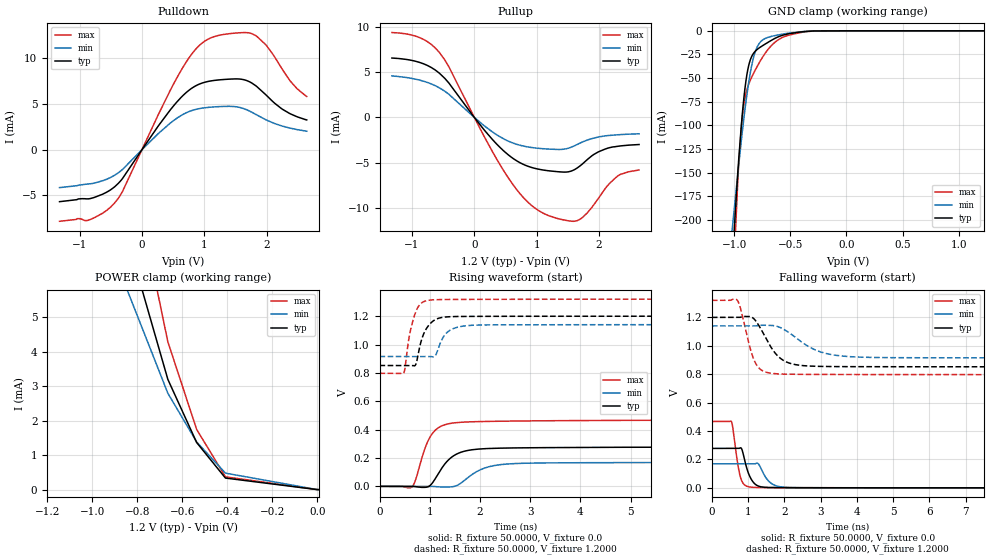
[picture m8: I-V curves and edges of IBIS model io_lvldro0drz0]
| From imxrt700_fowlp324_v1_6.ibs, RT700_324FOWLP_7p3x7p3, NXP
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[Model] io_lvldro0drz0
|   Model io_lvldro0drz0
| This model was characterised for following simulation conditions:
| External (pad) voltage:
|   - Typ: 1.2V,   - Min: 1.14V,   - Max: 1.32V
| Library cells for typ/min/max conditions are connected as defined below:
|  ipp_io - External Pad
|  ipp_do - Core Input
|  ipp_obe - Output Buffer Enable
|  config1v21v8 - vdd
|  drive0 - gnde
|  drive1 - gnde
|  gnd - gnd
|  gnde - gnde
|  ncgather - NC
|  vdd - vdd
|  vdde1v8 - vdde1v8
| All other pins connected to ground
Model_type I/O
Polarity   Non-Inverting
Enable   Active-Low
Vinl =   0.3600V
Vinh =   0.8400V
Vmeas =  0.6000V
Cref =   30.0000pF
Rref =   1.0000M
Vref =   1.2000V
C_comp   2.6161pF   2.5654pF   2.7101pF
|C_comp_pullup   1.3388pF   1.3968pF   1.2799pF
|C_comp_pulldown   0.0F   0.0F   0.0F
[Model Spec]
| variable   typ   min   max
Vinh   0.8400V   NA   NA
Vinl   0.3600V   NA   NA
Vref   1.8000V   1.8000V   1.8000V
Cref   30.0000pF   30.0000pF   30.0000pF
Rref   1.0000M   1.0000M   1.0000M
[Temperature Range]   25.0000   0.1250k   -40.0000
[Voltage Range]   1.2000V   1.1400V   1.3200V
[Pullup Reference]   1.2000V   1.1400V   1.3200V
[Pulldown Reference]   0.0V   0.0V   0.0V
[POWER Clamp Reference]   1.2000V   1.1400V   1.3200V
[GND Clamp Reference]   0.0V   0.0V   0.0V
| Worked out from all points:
|   slope of the pulldown table from 0 to 0.18 V, typ, clamps not added: 101 ohm
|   slope of the pullup table from 0 to 0.18 V, typ, clamps not added: 115 ohm
|   GND clamp passes 1 mA (typ) near -0.39 V on its own axis
|   POWER clamp passes 1 mA (typ) near -0.49 V on its own axis
|   rising waveform, R_fixture 50.0000, V_fixture 0.0: 20-80 % time 394ps typ, 485ps min, 296ps max; typ from 0 V to 0.278 V
|   rising waveform, R_fixture 50.0000, V_fixture 1.2000: 20-80 % time 204ps typ, 220ps min, 175ps max; typ from 0.852 V to 1.2 V
|   falling waveform, R_fixture 50.0000, V_fixture 0.0: 20-80 % time 218ps typ, 268ps min, 166ps max; typ from 0.278 V to 0 V
|   falling waveform, R_fixture 50.0000, V_fixture 1.2000: 20-80 % time 521ps typ, 847ps min, 323ps max; typ from 1.2 V to 0.852 V
[Pulldown]
|Voltage   I(typ)   I(min)   I(max)
-1.32V    -5.688mA   -4.151mA   -7.836mA
-856mV    -5.378mA   -3.749mA   -7.707mA
-440mV    -4.076mA   -2.805mA   -5.848mA
-312mV    -3.159mA   -2.166mA   -4.577mA
624mV     5.702mA    3.731mA    8.647mA
856mV     6.973mA    4.402mA    10.96mA
1.064V    7.478mA    4.635mA    12.12mA
1.568V    7.735mA    4.622mA    12.8mA
1.832V    6.962mA    3.837mA    12.46mA
1.992V    5.967mA    3.257mA    11.43mA
2.256V    4.407mA    2.573mA    8.725mA
2.64V     3.256mA    2.027mA    5.833mA
[Pullup]
|Voltage   I(typ)   I(min)   I(max)
-1.32V    6.575mA    4.592mA    9.394mA
-880mV    6.098mA    4.136mA    8.849mA
-560mV    4.9mA      3.277mA    7.198mA
-408mV    3.813mA    2.567mA    5.622mA
496mV     -3.862mA   -2.465mA   -6.171mA
792mV     -5.22mA    -3.183mA   -8.915mA
1.064V    -5.782mA   -3.445mA   -10.46mA
1.464V    -6.056mA   -3.485mA   -11.4mA
1.648V    -5.607mA   -3.003mA   -11.44mA
1.976V    -3.863mA   -2.192mA   -9.092mA
2.304V    -3.195mA   -1.922mA   -6.453mA
2.64V     -3.006mA   -1.816mA   -5.825mA
[GND_clamp]
|Voltage   I(typ)   I(min)   I(max)
-1.32V    -824mA     -526.2mA   -1.227A
-1.032V   -269.6mA   -225.5mA   -323.8mA
-968mV    -148.5mA   -150.4mA   -156.4mA
-936mV    -98.26mA   -114.7mA   -100.6mA
-920mV    -77.35mA   -98.01mA   -82.61mA
-880mV    -41.26mA   -61.23mA   -59.24mA
-856mV    -30.33mA   -43.55mA   -51.86mA
-816mV    -21.94mA   -23.19mA   -42.16mA
-744mV    -15.43mA   -9.413mA   -27.16mA
-584mV    -5.259mA   -3.813mA   -7.801mA
-352mV    -567.9uA   -545.2uA   -812.4uA
1.224V    19.17nA    663.1nA    12.5nA
[POWER_clamp]
|Voltage   I(typ)   I(min)   I(max)
-1.32V    19.77mA    14.89mA    27.18mA
-1.048V   11.92mA    9.166mA    16.41mA
-664mV    3.199mA    2.796mA    4.29mA
-536mV    1.366mA    1.383mA    1.747mA
-408mV    334.7uA    478.1uA    371.6uA
0V        17.28nA    129.7nA    13.53nA
8mV       16.9nA     117.4nA    13.43nA
[Ramp]
| variable   typ   min   max
dV/dt_r  0.1666/0.3936n   0.1014/0.4848n   0.2804/0.2955n
dV/dt_f  0.2087/0.5209n   0.1348/0.8462n   0.3138/0.3229n
R_load = 50.0000
[Rising Waveform]
R_fixture= 50.0000
V_fixture= 0.0
V_fixture_min= 0.0
V_fixture_max= 0.0
|time   V(typ)   V(min)   V(max)
0s        36.99nV    2.153uV    4.325nV
636.3ps   8.785uV    834.1nV    -6.706mV
715.1ps   -2.216mV   1.884uV    43.01mV
943.3ps   -5.366mV   -10.28uV   302.9mV
1.11ns    54.19mV    -1.954mV   395.8mV
1.474ns   215.3mV    -1.494mV   447mV
2.012ns   263.9mV    117.9mV    456.9mV
2.619ns   270.6mV    159.4mV    460.2mV
4.852ns   275.6mV    167.5mV    465.2mV
60ns      277.6mV    169.1mV    467.3mV
[Rising Waveform]
R_fixture= 50.0000
V_fixture= 1.2000
V_fixture_min= 1.1400
V_fixture_max= 1.3200
|time   V(typ)   V(min)   V(max)
0s        852.1mV    915.3mV    797mV
479.4ps   852.1mV    915.3mV    797.3mV
606.4ps   852.1mV    915.3mV    1.084V
741.2ps   881.8mV    915.3mV    1.247V
903.3ps   1.094V     915.3mV    1.306V
1.085ns   1.17V      913.6mV    1.315V
1.17ns    1.185V     971.1mV    1.317V
1.448ns   1.197V     1.109V     1.318V
2.199ns   1.199V     1.139V     1.319V
60ns      1.2V       1.14V      1.32V
[Falling Waveform]
R_fixture= 50.0000
V_fixture= 0.0
V_fixture_min= 0.0
V_fixture_max= 0.0
|time   V(typ)   V(min)   V(max)
0s        277.6mV    169.1mV    467.3mV
535.8ps   277.6mV    169.1mV    468.4mV
573.6ps   277.6mV    169mV      430mV
725.7ps   277.2mV    169mV      150mV
809.7ps   279.2mV    169mV      57.82mV
1.015ns   98.54mV    169mV      7.515mV
1.21ns    22.59mV    171.2mV    2.998mV
1.659ns   1.997mV    27.97mV    1.835mV
2.324ns   979.9uV    1.503mV    1.301mV
60ns      245.3nV    3.818uV    27.38nV
[Falling Waveform]
R_fixture= 50.0000
V_fixture= 1.2000
V_fixture_min= 1.1400
V_fixture_max= 1.3200
|time   V(typ)   V(min)   V(max)
0s        1.2V       1.14V      1.32V
697.5ps   1.2V       1.14V      1.322V
792.7ps   1.202V     1.14V      1.261V
1.084ns   1.203V     1.14V      957.1mV
1.227ns   1.17V      1.14V      867.9mV
1.676ns   972.3mV    1.143V     805.4mV
1.946ns   901.4mV    1.121V     800.8mV
3.066ns   854.6mV    951.6mV    798.3mV
4.595ns   852.8mV    917.4mV    797.6mV
60ns      852.1mV    915.3mV    797mV
